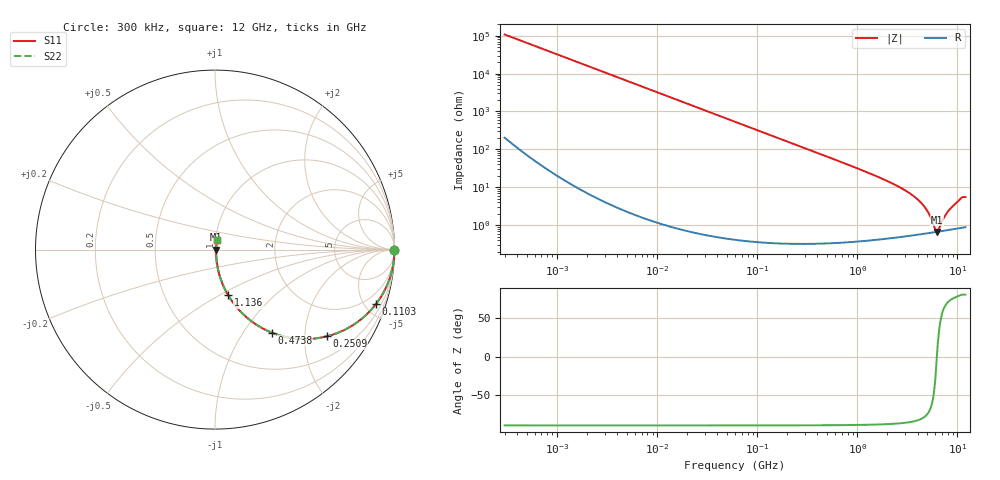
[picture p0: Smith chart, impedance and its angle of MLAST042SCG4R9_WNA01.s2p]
! MLAST042SCG4R9_WNA01  S-PARAMETER MODEL  ( General Type )
! Model Generated by TAIYO YUDEN Corporation (http://www.ty-top.com)
! Version 1.0
! TAIYO YUDEN Control No. 150820
! Copyright(c) 2015 TAIYO YUDEN CO.,LTD. All Rights Reserved.
! Product Description (link to TY-COMPAS)
! https://ds.yuden.co.jp/TYCOMPAS/or/detail?pn=MLAST042SCG4R9BWNA01&u=M
! Products Name : Multilayer Ceramic Capacitors
! Characteristics :
!  Capacitance : 4.9 pF , Rated Voltage : 25V , TCC : CG / C0G
!  Case Size : 0.4 x 0.2 / 0.016 x 0.008 [mm/inch] , Thickness : 0.2 / 0.008 [mm/inch]
!  (Conditions: Temperature = 25 degC , DC Bias Current/Voltage = 0A / 0V)
! External Node Assignments :
!  1  o---| |---o  2
! GND o---------o GND
! Frequency Range : 0.3MHz  -  12000MHz  [ 401 STEP ]
# MHz S RI R 50
! Freq[MHz].  S11 Real  S11 Imag  S21 Real  S21 Imag  S12 Real  S12 Imag  S22 Real  S22 Imag
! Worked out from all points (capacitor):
!   401 points, 300 kHz to 12 GHz, reference 50 ohm
!   read as one part in series: C = 4.92 pF near 316.3 kHz
!   lowest |Z| = 666 mohm at 6.188 GHz (marker M1)
!   series resonance near 6.222 GHz, so ESL is about 130 pH
!   S11 on the Smith chart (normalised r, x): 300 kHz: open; 110.3 MHz: 1.01, -5.87; 250.9 MHz: 1.01, -2.58; 473.8 MHz: 1.01, -1.36; 1.136 GHz: 1.01, -0.55; 12 GHz: 1.02, +0.11
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0.3  1 -0.000927  2.61e-06 0.000927  2.61e-06 0.000927  1 -0.000927
1.769972  1 -0.00547  3.24e-05 0.00547  3.24e-05 0.00547  1 -0.00547
10.44266  0.9989 -0.0322  0.00105 0.0322  0.00105 0.0322  0.9989 -0.0322
60  0.9667 -0.1791  0.0333 0.1791  0.0333 0.1791  0.9667 -0.1791
110.3493  0.8956 -0.3052  0.1044 0.3052  0.1044 0.3052  0.8956 -0.3052
164.1901  0.7948 -0.403  0.2052 0.403  0.2052 0.403  0.7948 -0.403
250.8588  0.6238 -0.4832  0.3762 0.4832  0.3762 0.4832  0.6238 -0.4832
353.9943  0.454 -0.4961  0.546 0.4961  0.546 0.4961  0.454 -0.4961
473.7541  0.3167 -0.4628  0.6833 0.4628  0.6833 0.4628  0.3167 -0.4628
723.8279  0.1649 -0.3672  0.8351 0.3672  0.8351 0.3672  0.1649 -0.3672
1135.593  0.0736 -0.2544  0.9264 0.2544  0.9264 0.2544  0.0736 -0.2544
2088.533  0.0228 -0.1338  0.9772 0.1338  0.9772 0.1338  0.0228 -0.1338
3190.978  0.0106 -0.0736  0.9894 0.0736  0.9894 0.0736  0.0106 -0.0736
4270.516  0.00728 -0.0396  0.9927 0.0396  0.9927 0.0396  0.00728 -0.0396
5006.236  0.00657 -0.0226  0.9934 0.0226  0.9934 0.0226  0.00657 -0.0226
5868.704  0.00649 -0.00605  0.9935 0.00605  0.9935 0.00605  0.00649 -0.00605
6188.031  0.00659 -0.000507  0.9934 0.000507  0.9934 0.000507  0.00659 -0.000507
6524.734  0.00676 0.00416  0.9932 -0.00416  0.9932 -0.00416  0.00676 0.00416
7448.838  0.00735 0.0151  0.9926 -0.0151  0.9926 -0.0151  0.00735 0.0151
8503.825  0.00821 0.0259  0.9918 -0.0259  0.9918 -0.0259  0.00821 0.0259
10793.46  0.0107 0.0485  0.9893 -0.0485  0.9893 -0.0485  0.0107 0.0485
12000  0.0117 0.0535  0.9883 -0.0535  0.9883 -0.0535  0.0117 0.0535
